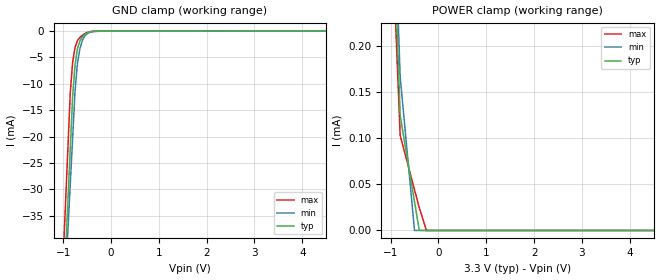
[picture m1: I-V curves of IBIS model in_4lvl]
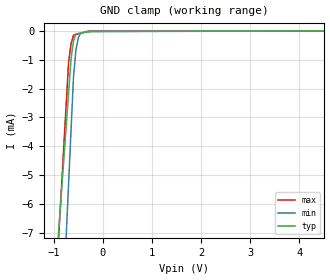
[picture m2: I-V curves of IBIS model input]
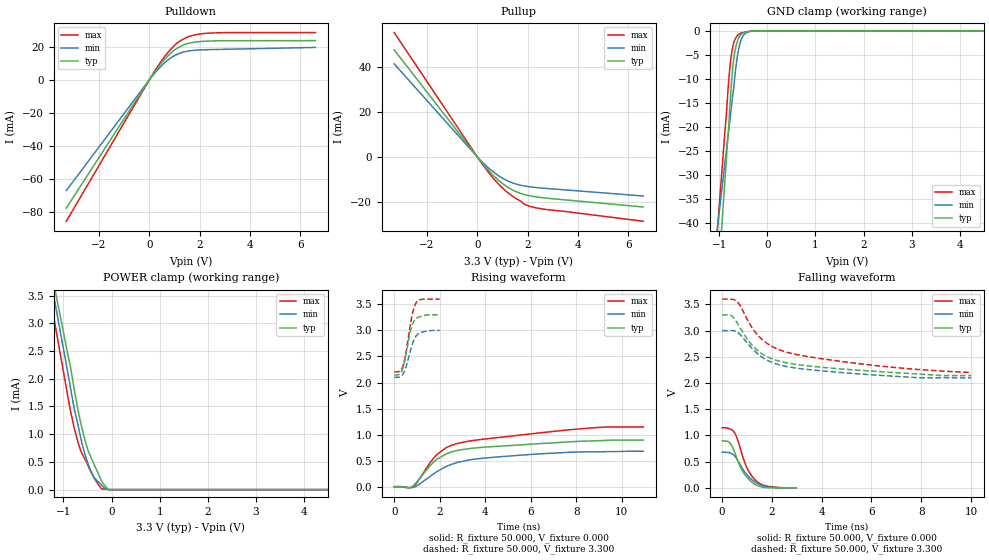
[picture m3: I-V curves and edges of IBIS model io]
[IBIS Ver]   3.2
[Comment Char] |_char
[File Name]   pcm1681pwp.ibs
[File Rev]   3.0
[Source]
| This model file was created by Teraspeed Consulting Group LLC
| (http://www.teraspeed.com/).
[Date]   06-19-2008
[Notes]   Quality Check of this IBIS model: Model Passes IBIS Check
   Model parses into ICX IS. Simulation done with Hyperlynx.
   1. MIN TYP MAX information is based on Temprature and Voltage
   characteristics only.
[Disclaimer]
| This model is designed as an aid for customers of Texas Instruments.
| TI and its licensors and suppliers make no warranties, either expressed
| or implied, with respect to this  model, including the warranties of
| merchantability or fitness for a particular purpose.
| The model is provided solely on an "as is" basis. The entire risk as to
| its quality and performance is with the customer.
[Copyright]
| (C) Copyright 2008 Texas Instruments Incorporated. All rights reserved.
[Component]   PCM1681PWP
[Manufacturer] TI
[Package]
| variable   typ   min   max
R_pkg  1.820E-01   1.700E-01   1.940E-01
L_pkg  4.420E-09   2.800E-09   6.040E-09
C_pkg  7.530E-13   6.210E-13   8.850E-13
[Pin] signal_name  model_name  R_pin  L_pin C_pin
1   ZR1/ZR1/FMT0 io   1.940E-01   6.040E-09   8.850E-13
2   _MS/ADR/FMT1 input   1.900E-01   5.500E-09   8.410E-13
3   MC/SCL/DEMP  input   1.860E-01   4.960E-09   7.970E-13
4   MD/SDA/MUTE  io_od   1.820E-01   4.420E-09   7.530E-13
5   SCK   input   1.780E-01   3.880E-09   7.090E-13
6   DATA1   input   1.740E-01   3.340E-09   6.650E-13
7   BCK   input   1.700E-01   2.800E-09   6.210E-13
8   LRCK   input   1.700E-01   2.800E-09   6.210E-13
9   VDD   POWER   1.740E-01   3.340E-09   6.650E-13
10   DGND   GND   1.780E-01   3.880E-09   7.090E-13
11   DATA2   input   1.820E-01   4.420E-09   7.530E-13
12   DATA3   input   1.860E-01   4.960E-09   7.970E-13
13   DATA4   input   1.900E-01   5.500E-09   8.410E-13
14   MSEL   in_4lvl  1.940E-01   6.040E-09   8.850E-13
15   VOUT8   term   1.940E-01   6.040E-09   8.850E-13
16   VOUT7   term   1.900E-01   5.500E-09   8.410E-13
17   VCC1   POWER   1.860E-01   4.960E-09   7.970E-13
18   AGND1   GND   1.820E-01   4.420E-09   7.530E-13
19   VOUT6   term   1.780E-01   3.880E-09   7.090E-13
20   VOUT5   term   1.740E-01   3.340E-09   6.650E-13
21   VOUT4   term   1.700E-01   2.800E-09   6.210E-13
22   VOUT3   term   1.700E-01   2.800E-09   6.210E-13
23   VCC2   POWER   1.740E-01   3.340E-09   6.650E-13
24   AGND2   GND   1.780E-01   3.880E-09   7.090E-13
25   VCOM   term   1.820E-01   4.420E-09   7.530E-13
26   VOUT2   term   1.860E-01   4.960E-09   7.970E-13
27   VOUT1   term   1.900E-01   5.500E-09   8.410E-13
28   ZR2   output   1.940E-01   6.040E-09   8.850E-13
[Model] term
Model_type Terminator
C_comp   0  0  0
| variable   typ   min   max
[Voltage Range]   5.00000V  4.75000V  5.25000V
[POWER Clamp Reference]  5.00000V  4.75000V  5.25000V
[GND Clamp Reference]   0.00000V  0.00000V  0.00000V
[Temperature Range]   25   85   -40
| Models and submodels in the file (6): term (Terminator), in_4lvl (Input), input (Input), io (I/O), io_od (I/O_open_drain), output (Output)
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[Model] in_4lvl
Model_type Input
Vinl = 800.000mV
Vinh = 2.00000V
C_comp 447.0fF  447.0fF  447.0fF
| variable typ   min   max
[Voltage Range] 3.30000V 3.00000V 3.60000V
[POWER Clamp Reference] 3.30000V 3.00000V 3.60000V
[GND Clamp Reference] 0.00000V 0.00000V 0.00000V
[Temperature Range]   25   85   -40
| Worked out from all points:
|   GND clamp passes 1 mA (typ) near -0.59 V on its own axis
[GND Clamp]
-3.3V     -515.3mA   -464.1mA   -530.6mA
-850mV    -22.33mA   -29.06mA   -11.68mA
-800mV    -12.27mA   -20.18mA   -5.881mA
-750mV    -6.358mA   -11.3mA    -3.083mA
-700mV    -3.327mA   -6.091mA   -1.811mA
-650mV    -1.913mA   -3.432mA   -1.213mA
-600mV    -1.088mA   -1.825mA   -797uA
-550mV    -638uA     -975.9uA   -530.8uA
-500mV    -366.4uA   -524.9uA   -264.6uA
-350mV    -65.97uA   -54.63uA   -41.27uA
-175mV    -20.2uA    -18.01uA   -20.96uA
6.6V      70.42uA    94.98uA    69.4uA
[POWER Clamp]
-3.3V     3.852mA    3.942mA    3.685mA
-1.15V    646.5uA    695.2uA    550.2uA
-800mV    124.7uA    166.7uA    103uA
-575mV    54.55uA    41.66uA    58.87uA
-500mV    31.17uA    0A         44.15uA
-400mV    0A         0A         24.53uA
-250mV    0A         0A         0A
6.6V      0A         0A         0A
[Model] input
Model_type Input
Vinl = 800.000mV
Vinh = 2.00000V
C_comp 621.0fF  621.0fF  621.0fF
| variable typ   min   max
[Voltage Range] 3.30000V 3.00000V 3.60000V
[POWER Clamp Reference] 3.30000V 3.00000V 3.60000V
[GND Clamp Reference] 0.00000V 0.00000V 0.00000V
[Temperature Range]   25   85   -40
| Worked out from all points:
|   GND clamp passes 1 mA (typ) near -0.65 V on its own axis
[GND Clamp]
-3.3V     -63.83mA   -101.9mA   -79.25mA
-700mV    -2.156mA   -5.322mA   -1.079mA
-650mV    -970.2uA   -3.465mA   -451.1uA
-600mV    -347.4uA   -1.607mA   -147.9uA
-550mV    -99.42uA   -655.3uA   -124.6uA
-500mV    -85.4uA    -227.4uA   -101.2uA
-450mV    -71.38uA   -63.1uA    -77.89uA
-300mV    -29.31uA   -30.65uA   -7.836uA
-275mV    -22.3uA    -25.24uA   -7.789uA
-225mV    -22.04uA   -14.43uA   -7.694uA
6.6V      13.26uA    11.26uA    5.18uA
[POWER Clamp]
-3.3V     0A         0A         0A
6.6V      0A         0A         0A
[Model]   io
Model_type I/O
Vinl=8.000E-01
Vinh=2.000E+00
Vref=0.000E+00
Rref=1.000E+06
Cref=0.000E+00
Vmeas=1.650E+00
C_comp   648.0fF   648.0fF   648.0fF
[Voltage Range]   3.300E+00   3.000E+00   3.600E+00
[POWER Clamp Reference]   3.300E+00   3.000E+00   3.600E+00
[GND Clamp Reference]   0.000E+00   0.000E+00   0.000E+00
[Pullup Reference]   3.300E+00   3.000E+00   3.600E+00
[Pulldown Reference]   0.000E+00   0.000E+00   0.000E+00
[Temperature Range]   25   85   -40
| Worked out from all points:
|   slope of the pulldown table from 0 to 0.495 V, typ, clamps not added: 47.9 ohm
|   slope of the pullup table from 0 to 0.495 V, typ, clamps not added: 75 ohm
|   GND clamp passes 1 mA (typ) near -0.57 V on its own axis
|   POWER clamp passes 1 mA (typ) near -0.58 V on its own axis
|   rising waveform, R_fixture 50.000, V_fixture 0.000: 20-80 % time 1.91ns typ, 2.48ns min, 2.79ns max; typ from 0 V to 0.895 V
|   falling waveform, R_fixture 50.000, V_fixture 0.000: 20-80 % time 570ps typ, 656ps min, 566ps max; typ from 0.895 V to 0 V
|   rising waveform, R_fixture 50.000, V_fixture 3.300: 20-80 % time 329ps typ, 362ps min, 321ps max; typ from 2.14 V to 3.3 V
|   falling waveform, R_fixture 50.000, V_fixture 3.300: 20-80 % time 2.02ns typ, 2.14ns min, 2.82ns max; typ from 3.3 V to 2.14 V
[GND Clamp]
-3.3V     -385.7mA   -236.3mA   -336.8mA
-880mV    -30.73mA   -27.26mA   -20.59mA
-800mV    -19.42mA   -20.35mA   -9.852mA
-780mV    -15.87mA   -18.62mA   -7.632mA
-740mV    -9.961mA   -15.16mA   -4.443mA
-720mV    -7.709mA   -13.43mA   -3.354mA
-660mV    -3.514mA   -7.992mA   -1.511mA
-620mV    -2.074mA   -5.051mA   -956.6uA
-560mV    -886.6uA   -2.284mA   -532.8uA
-440mV    -233.2uA   -396.9uA   -223.7uA
-280mV    0A         0A         0A
6.6V      0A         0A         0A
[Power Clamp]
-3.3V     12.83mA    13.4mA     13.34mA
-960mV    2.667mA    2.35mA     1.931mA
-900mV    2.393mA    2.064mA    1.638mA
-860mV    2.248mA    1.866mA    1.451mA
-760mV    1.731mA    1.402mA    1.057mA
-640mV    1.201mA    930.3uA    700.9uA
-580mV    984.6uA    720.8uA    594.8uA
-480mV    684.7uA    443.6uA    416.2uA
-360mV    448.8uA    211.8uA    202.8uA
-200mV    149.3uA    74.96uA    12.57uA
-60mV     0A         0A         0A
6.6V      0A         0A         0A
[Pullup]
-3.3V     47.49mA    41.29mA    55.2mA
180mV     -2.565mA   -2.087mA   -2.929mA
740mV     -9.368mA   -7.553mA   -10.81mA
1.06V     -12.33mA   -9.836mA   -14.46mA
1.3V      -14.1mA    -11.15mA   -16.68mA
1.74V     -16.33mA   -12.67mA   -19.79mA
1.84V     -16.66mA   -12.89mA   -20.9mA
2.34V     -17.8mA    -13.65mA   -22.68mA
6.6V      -22.3mA    -17.41mA   -28.65mA
[Pulldown]
-3.3V     -77.4mA    -66.86mA   -85.34mA
140mV     3.167mA    2.696mA    3.525mA
620mV     12.54mA    10.43mA    14.23mA
920mV     17.01mA    13.85mA    19.51mA
1.1V      18.97mA    15.3mA     22.02mA
1.5V      21.72mA    17.19mA    25.66mA
1.9V      22.83mA    17.86mA    27.34mA
2.2V      23.2mA     18.08mA    27.92mA
3.06V     23.53mA    18.38mA    28.44mA
6.6V      23.6mA     19.49mA    28.45mA
[Rising Waveform]
R_fixture = 50.000
V_fixture = 0.000
V_fixture_min = 0.000
V_fixture_max = 0.000
|  time   V(typ)   V(min)   V(max)
0s        0V         0V         0V
600ps     -22.83mV   -16.36mV   -17.51mV
840ps     19.05mV    -12.14mV   2.184mV
1.56ns    396.8mV    190.8mV    452mV
1.89ns    530.1mV    292.5mV    621.3mV
2.33ns    637.8mV    395.7mV    758.1mV
2.86ns    703.1mV    473.8mV    838.5mV
3.98ns    759mV      549.9mV    914.7mV
7.91ns    865.9mV    663.7mV    1.101V
10.95ns   895.1mV    681.1mV    1.146V
[Falling Waveform]
R_fixture = 50.000
V_fixture = 0.000
V_fixture_min = 0.000
V_fixture_max = 0.000
|  time   V(typ)   V(min)   V(max)
0s        895.1mV    681.1mV    1.146V
280ps     870.6mV    672.2mV    1.129V
500ps     681.2mV    609.5mV    1.052V
610ps     541mV      536.2mV    936mV
810ps     327.2mV    374.7mV    622.8mV
980ps     212.1mV    258.8mV    399.8mV
1.18ns    117.1mV    163.2mV    234.9mV
1.39ns    50.56mV    93.46mV    125mV
1.83ns    1.468mV    19.58mV    31.4mV
2.96ns    0V         0V         0V
[Rising Waveform]
R_fixture = 50.000
V_fixture = 3.300
V_fixture_min = 3.000
V_fixture_max = 3.600
|  time   V(typ)   V(min)   V(max)
0s        2.142V     2.099V     2.204V
250ps     2.164V     2.109V     2.22V
390ps     2.291V     2.164V     2.322V
520ps     2.545V     2.298V     2.576V
720ps     2.996V     2.623V     3.133V
790ps     3.102V     2.729V     3.298V
870ps     3.18V      2.823V     3.436V
970ps     3.23V      2.898V     3.537V
1.18ns    3.27V      2.96V      3.595V
2ns       3.3V       3V         3.6V
[Falling Waveform]
R_fixture = 50.000
V_fixture = 3.300
V_fixture_min = 3.000
V_fixture_max = 3.600
|  time   V(typ)   V(min)   V(max)
0s        3.3V       3V         3.6V
380ps     3.281V     3.002V     3.597V
580ps     3.167V     2.981V     3.568V
730ps     3.044V     2.923V     3.476V
1.02ns    2.828V     2.759V     3.202V
1.5ns     2.591V     2.529V     2.877V
1.95ns    2.471V     2.403V     2.712V
2.6ns     2.384V     2.313V     2.587V
6.22ns    2.221V     2.15V      2.33V
10.01ns   2.142V     2.099V     2.204V
[Ramp]
dV/dt_r   5.2957E-01/1.8780E-09   4.0232E-01/2.4679E-09   6.7583E-01/2.8000E-09
dV/dt_f   6.9475E-01/2.0178E-09   5.4036E-01/2.1344E-09   8.3763E-01/2.8124E-09
R_load = 50
